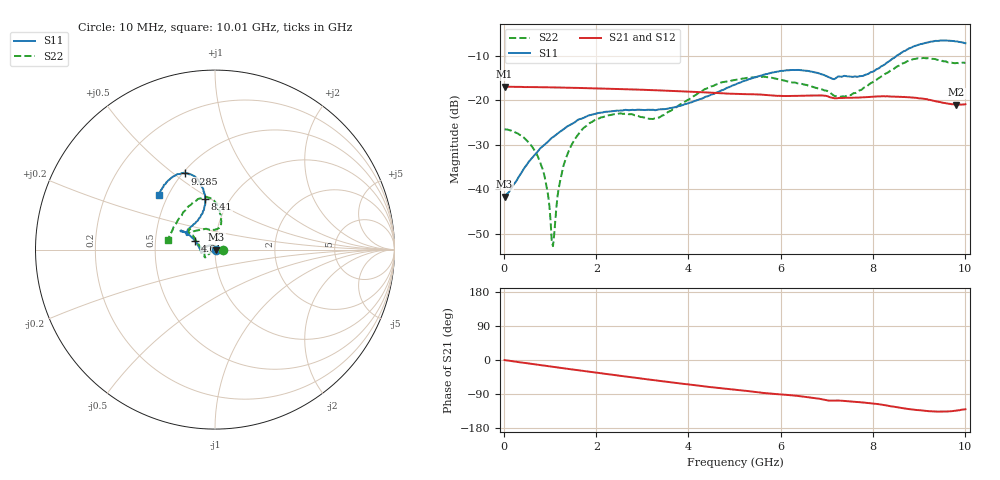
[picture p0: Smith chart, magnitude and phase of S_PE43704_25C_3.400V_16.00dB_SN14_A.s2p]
! Device ID: PE43704
! Dir: z:\PE43704\PE43704_Char_1_20130516\PE43704\AMB\3p400V\16p00dB
! Serial: 14
! Insertion: A
! Impedance: 50 ohm
! Temp: Amb
! VDD: 3.400V
! Attenuation Step: 16.00dB
! IDD: 1.139512e-01mA
#  Hz  S  RI  R  50
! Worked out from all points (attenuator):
!   401 points, 10 MHz to 10.01 GHz, reference 50 ohm
!   highest |S21| = -16.95 dB at 10 MHz (marker M1); lowest = -21.0 dB at 9.81 GHz (marker M2)
!   lowest |S11| = -41.7 dB at 10 MHz (marker M3), VSWR 1.02, Z = 50.8 + j0.0372 ohm
!   |S11| at or under -10 dB: start of sweep to 8.522 GHz
!   |S22| runs from -52.8 to -10.5 dB; largest |S21 - S12| = 0.0017
!   S11 on the Smith chart (normalised r, x): 10 MHz: 1.02, +0.00; 4.61 GHz: 0.79, +0.08; 8.41 GHz: 0.77, +0.48; 9.285 GHz: 0.51, +0.55; 10.01 GHz: 0.45, +0.34
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1e7  0.00826 0.000366  0.142 -0.00046  0.142 -0.000475  0.0472 6.44e-07
4.1e8  0.00211 0.0163  0.1397 -0.0178  0.1398 -0.0174  0.0384 0.0055
7.1e8  -0.0105 0.0237  0.1373 -0.0295  0.1372 -0.0295  0.024 0.00556
8.85e8  -0.0201 0.0248  0.1351 -0.0364  0.1351 -0.0363  0.013 0.00294
1.01e9  -0.0275 0.0246  0.1335 -0.0412  0.1334 -0.0411  0.0042 -0.000121
1.06e9  -0.0304 0.0237  0.1328 -0.0431  0.1328 -0.043  0.000738 -0.00218
1.21e9  -0.0387 0.0211  0.1303 -0.0487  0.1302 -0.0487  -0.00952 -0.00734
1.31e9  -0.0443 0.0189  0.1283 -0.0523  0.1284 -0.0523  -0.0165 -0.0113
1.685e9  -0.0619 0.00645  0.1208 -0.0652  0.1208 -0.0651  -0.0372 -0.0279
2.36e9  -0.0742 -0.0142  0.1041 -0.0848  0.1042 -0.0849  -0.0542 -0.0432
3.36e9  -0.0783 -0.0108  0.0742 -0.1056  0.0743 -0.1056  -0.0635 -0.0076
4.61e9  -0.112 0.0496  0.0344 -0.1159  0.0347 -0.1157  -0.1273 0.0811
5.01e9  -0.1319 0.071  0.0237 -0.1157  0.0237 -0.1158  -0.1418 0.0921
5.96e9  -0.1836 0.1047  -0.00081 -0.1123  -0.00042 -0.1122  -0.1335 0.1076
6.685e9  -0.1844 0.0998  -0.0188 -0.1116  -0.0189 -0.1115  -0.0928 0.1079
7.385e9  -0.1516 0.1112  -0.0331 -0.1016  -0.033 -0.1012  -0.00361 0.1102
7.835e9  -0.0911 0.1703  -0.0418 -0.0999  -0.0417 -0.0998  0.0316 0.1374
8.36e9  -0.0544 0.27  -0.0573 -0.0944  -0.0574 -0.0949  0.0278 0.2089
8.41e9  -0.0549 0.2835  -0.0587 -0.093  -0.0587 -0.0936  0.0226 0.2183
9.285e9  -0.1665 0.424  -0.0716 -0.0697  -0.0714 -0.0694  -0.1044 0.2728
9.81e9  -0.2793 0.3635  -0.0616 -0.0647  -0.0618 -0.0642  -0.2248 0.1338
1.001e10  -0.312 0.3063  -0.058 -0.0693  -0.0596 -0.0698  -0.2609 0.0508
